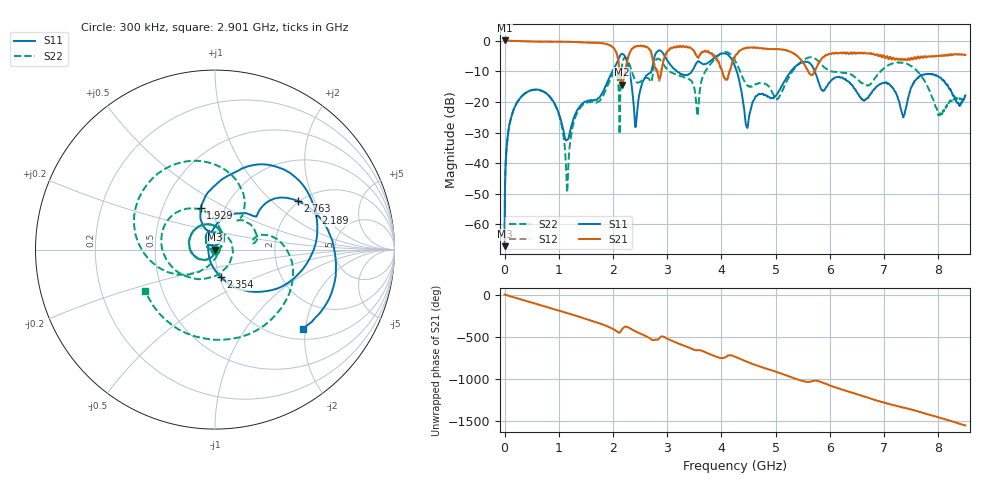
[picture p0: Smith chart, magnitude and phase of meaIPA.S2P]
!Agilent Technologies,E5071B,MY42402595,A.08.01
!Date: Mon Jan 01 23:33:36 2001
!Data & Calibration Information:
!Freq	S11:SOLT2(ON)	S21:SOLT2(ON)	S12:SOLT2(ON)	S22:SOLT2(ON)
# Hz S dB R 50
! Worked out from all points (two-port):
!   1601 points, 300 kHz to 8.5 GHz, reference 50 ohm
!   highest |S21| = 0.04 dB at 300 kHz (marker M1); lowest = -14.3 dB at 2.157 GHz (marker M2)
!   |S21| within 3 dB of the highest: start of sweep to 2.034 GHz; 4.37 GHz to 5.143 GHz (773.8 MHz wide, 16.3 % of centre)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
!   lowest |S11| = -67.1 dB at 300 kHz (marker M3), VSWR 1.00, Z = 50 + j0.00459 ohm
!   |S11| at or under -10 dB: start of sweep to 1.99 GHz; 4.281 GHz to 5.282 GHz (1 GHz wide, 20.9 % of centre); 5.72 GHz to end of sweep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
!   |S22| runs from -64.5 to -3.7 dB; largest |S21 - S12| = 0.068
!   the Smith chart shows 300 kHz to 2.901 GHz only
!   S11 on the Smith chart (normalised r, x): 300 kHz: 1.00, +0.00; 1.929 GHz: 0.77, +0.38; 2.189 GHz: 2.76, +1.73; 2.354 GHz: 1.02, -0.32; 2.763 GHz: 1.96, +1.49; 2.901 GHz: 1.24, -1.95
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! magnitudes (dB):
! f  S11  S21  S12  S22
! 300 kHz  -67.1  0.0  0.0  -64.5
! 74.67 MHz  -28.9  0.0  -0.1  -28.9
! 271.2 MHz  -19.2  -0.2  -0.2  -19.1
! 882.1 MHz  -19.4  -0.4  -0.3  -19.5
! 1.153 GHz  -32.4  -0.4  -0.4  -49.6
! 1.419 GHz  -20.8  -0.6  -0.6  -21.4
! 1.929 GHz  -12.3  -1.4  -1.5  -13.5
! 2.157 GHz  -4.3  -14.3  -14.2  -9.5
! 2.189 GHz  -4.5  -13.0  -13.2  -6.2
! 2.354 GHz  -16.1  -2.7  -2.7  -10.4
! 2.428 GHz  -26.5  -2.0  -1.9  -13.4
! 2.763 GHz  -5.4  -8.3  -7.8  -7.6
! 2.837 GHz  -3.3  -11.8  -11.2  -5.9
! 2.901 GHz  -3.6  -9.2  -9.0  -6.9
! 3.554 GHz  -7.0  -5.3  -5.3  -24.3
! 4.25 GHz  -8.4  -5.2  -5.3  -6.5
! 4.473 GHz  -28.3  -2.3  -2.4  -14.6
! 5.669 GHz  -8.2  -11.3  -11.3  -5.5
! 7.087 GHz  -14.1  -6.1  -5.4  -8.0
! 7.353 GHz  -25.1  -6.2  -6.2  -7.3
! 7.708 GHz  -11.2  -5.5  -5.7  -12.0
! 8.5 GHz  -17.9  -4.6  -4.7  -20.4
